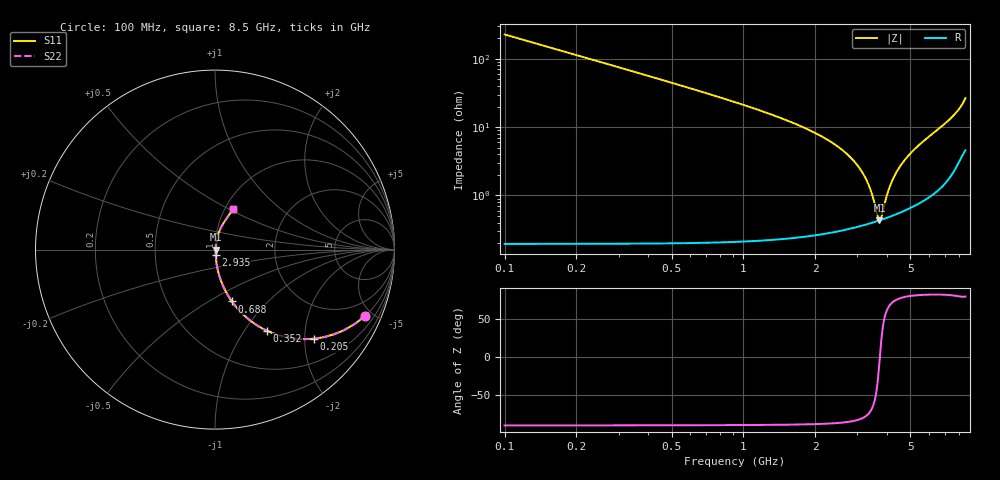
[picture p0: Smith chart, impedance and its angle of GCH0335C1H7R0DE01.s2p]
!Murata Part Number: GCH0335C1H7R0DE01
!These Parameters are Measured in Series Mode Connection
!Data Generated on Mar 13, 2026
!  o--ll--o
!Port1  Port2
!  o------o
!Operation Temp=25[degC], DC Bias Voltage=0[V]
!Freq. Start=100[MHz] Stop=9[GHz] 401[Steps]
# Hz S RI R 50
!Freq.(Hz) S11(Real) S11(Imag) S21(Real) S21(Imag) S12(Real) S12(Imag) S22(Real) S22(Imag)
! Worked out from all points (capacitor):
!   401 points, 100 MHz to 8.5 GHz, reference 50 ohm
!   read as one part in series: C = 7 pF near 142 MHz
!   lowest |Z| = 434 mohm at 3.712 GHz (marker M1)
!   series resonance near 3.725 GHz, so ESL is about 260 pH
!   S11 on the Smith chart (normalised r, x): 100 MHz: 1.00, -4.54; 205 MHz: 1.00, -2.21; 352 MHz: 1.00, -1.28; 688 MHz: 1.00, -0.64; 2.935 GHz: 1.01, -0.06; 8.5 GHz: 1.09, +0.52
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1e8  0.8375 -0.3685  0.1625 0.3685  0.1625 0.3685  0.8375 -0.3685
2.05e8  0.5501 -0.4966  0.4499 0.4966  0.4499 0.4966  0.5501 -0.4966
3.52e8  0.2914 -0.4529  0.7086 0.4529  0.7086 0.4529  0.2914 -0.4529
4.99e8  0.1681 -0.3718  0.8319 0.3718  0.8319 0.3718  0.1681 -0.3718
6.88e8  0.0942 -0.289  0.9058 0.289  0.9058 0.289  0.0942 -0.289
1.045e9  0.0408 -0.1925  0.9592 0.1925  0.9592 0.1925  0.0408 -0.1925
1.507e9  0.0181 -0.1245  0.9819 0.1245  0.9819 0.1245  0.0181 -0.1245
2.41e9  0.006 -0.0554  0.994 0.0554  0.994 0.0554  0.006 -0.0554
2.914e9  0.00432 -0.0309  0.9957 0.0309  0.9957 0.0309  0.00432 -0.0309
2.935e9  0.00429 -0.03  0.9957 0.03  0.9957 0.03  0.00429 -0.03
3.334e9  0.00402 -0.014  0.996 0.014  0.996 0.014  0.00402 -0.014
3.481e9  0.00407 -0.00857  0.9959 0.00857  0.9959 0.00857  0.00407 -0.00857
3.649e9  0.00422 -0.00261  0.9958 0.00261  0.9958 0.00261  0.00422 -0.00261
3.712e9  0.00429 -0.000437  0.9957 0.000437  0.9957 0.000437  0.00429 -0.000437
3.775e9  0.00438 0.00171  0.9956 -0.00171  0.9956 -0.00171  0.00438 0.00171
4.048e9  0.00489 0.0107  0.9951 -0.0107  0.9951 -0.0107  0.00489 0.0107
4.3e9  0.00553 0.0187  0.9945 -0.0187  0.9945 -0.0187  0.00553 0.0187
4.867e9  0.00754 0.036  0.9925 -0.036  0.9925 -0.036  0.00754 0.036
5.707e9  0.0122 0.0616  0.9878 -0.0616  0.9878 -0.0616  0.0122 0.0616
7.114e9  0.0291 0.1133  0.9709 -0.1133  0.9709 -0.1133  0.0291 0.1133
7.975e9  0.0582 0.1643  0.9418 -0.1643  0.9418 -0.1643  0.0582 0.1643
8.5e9  0.1001 0.2254  0.8999 -0.2254  0.8999 -0.2254  0.1001 0.2254
